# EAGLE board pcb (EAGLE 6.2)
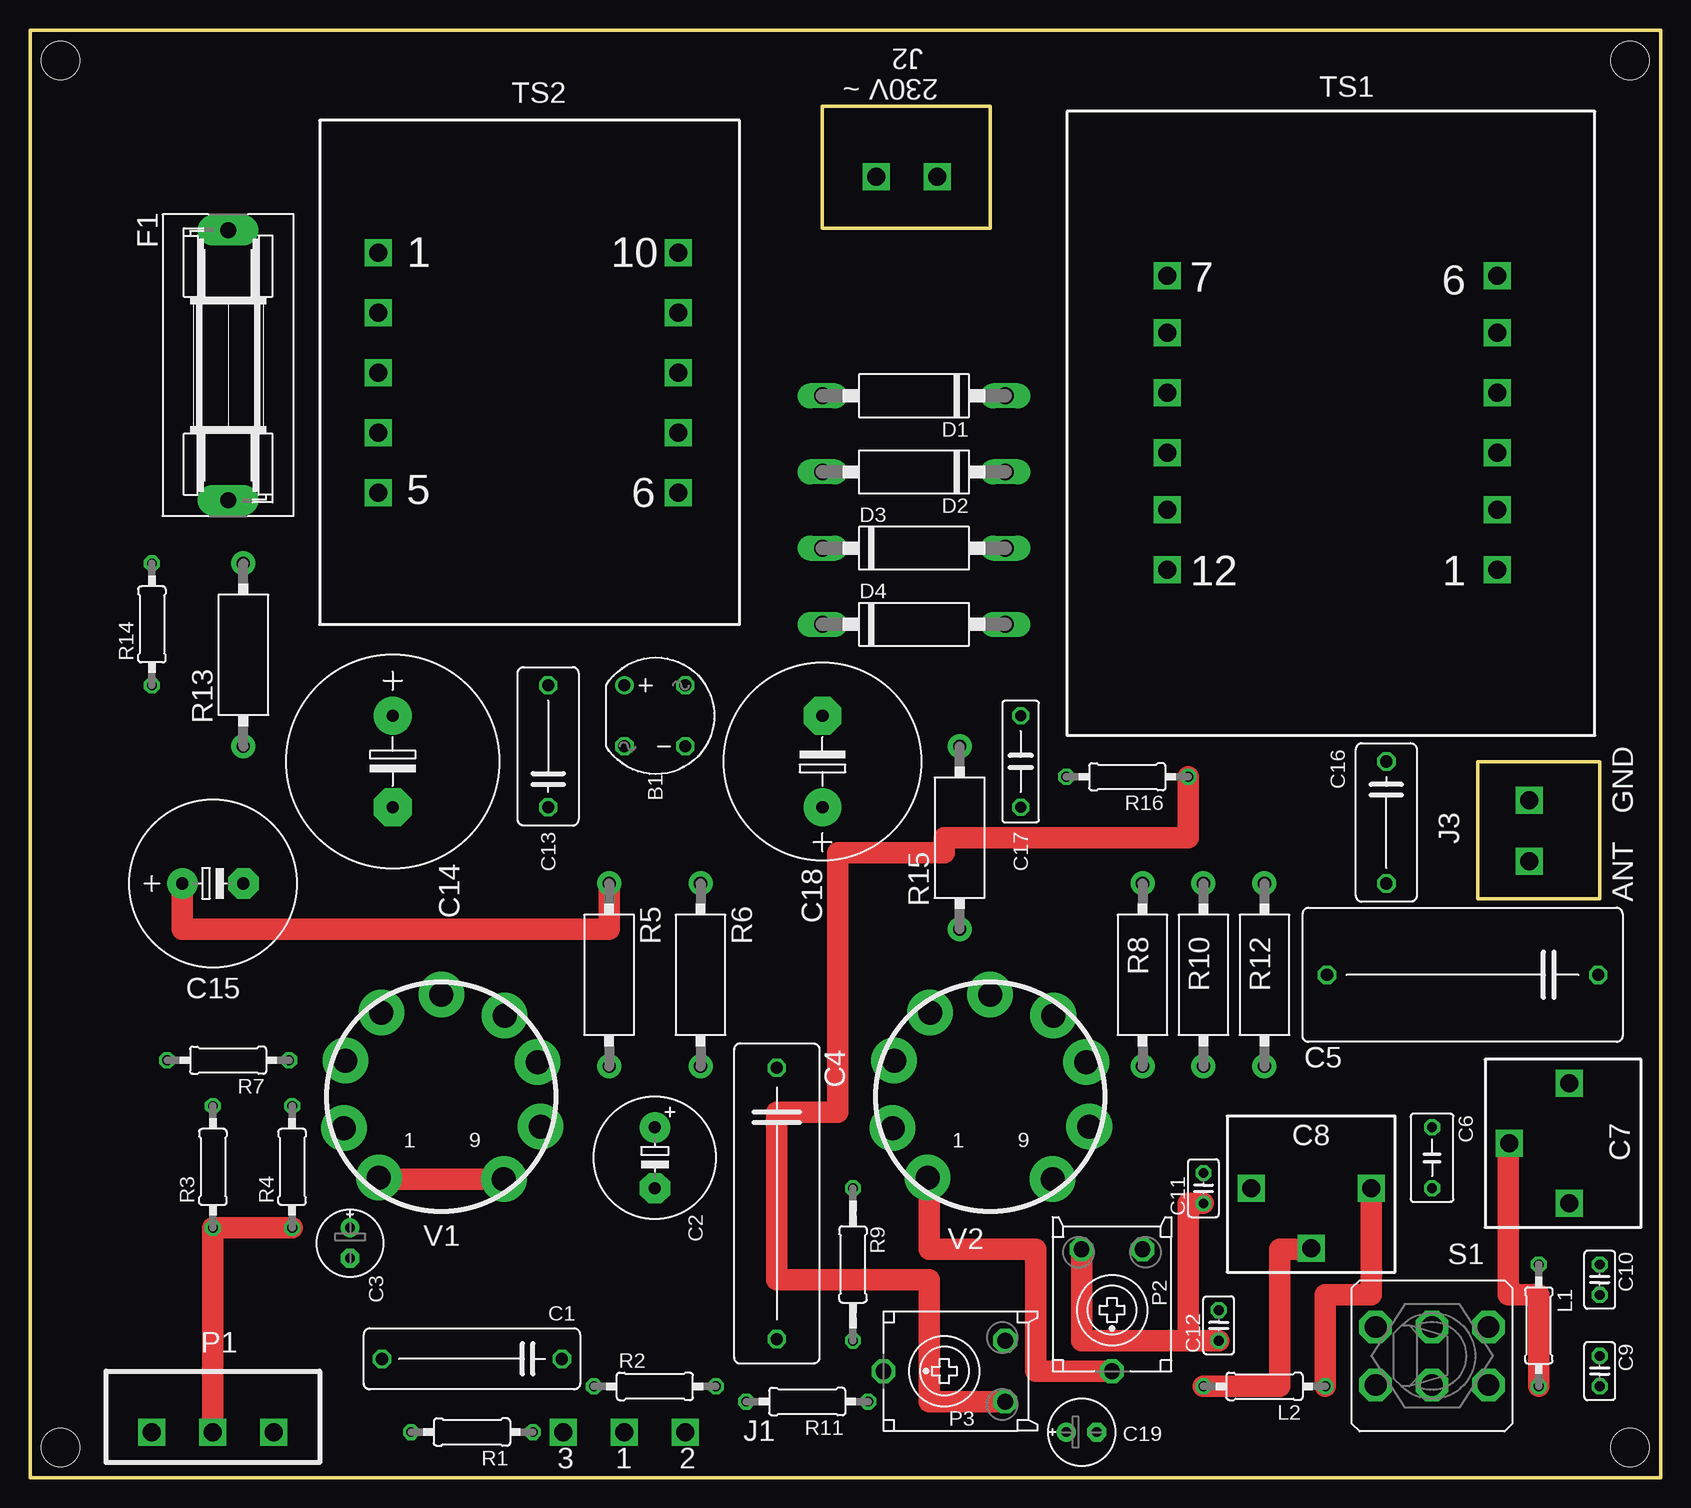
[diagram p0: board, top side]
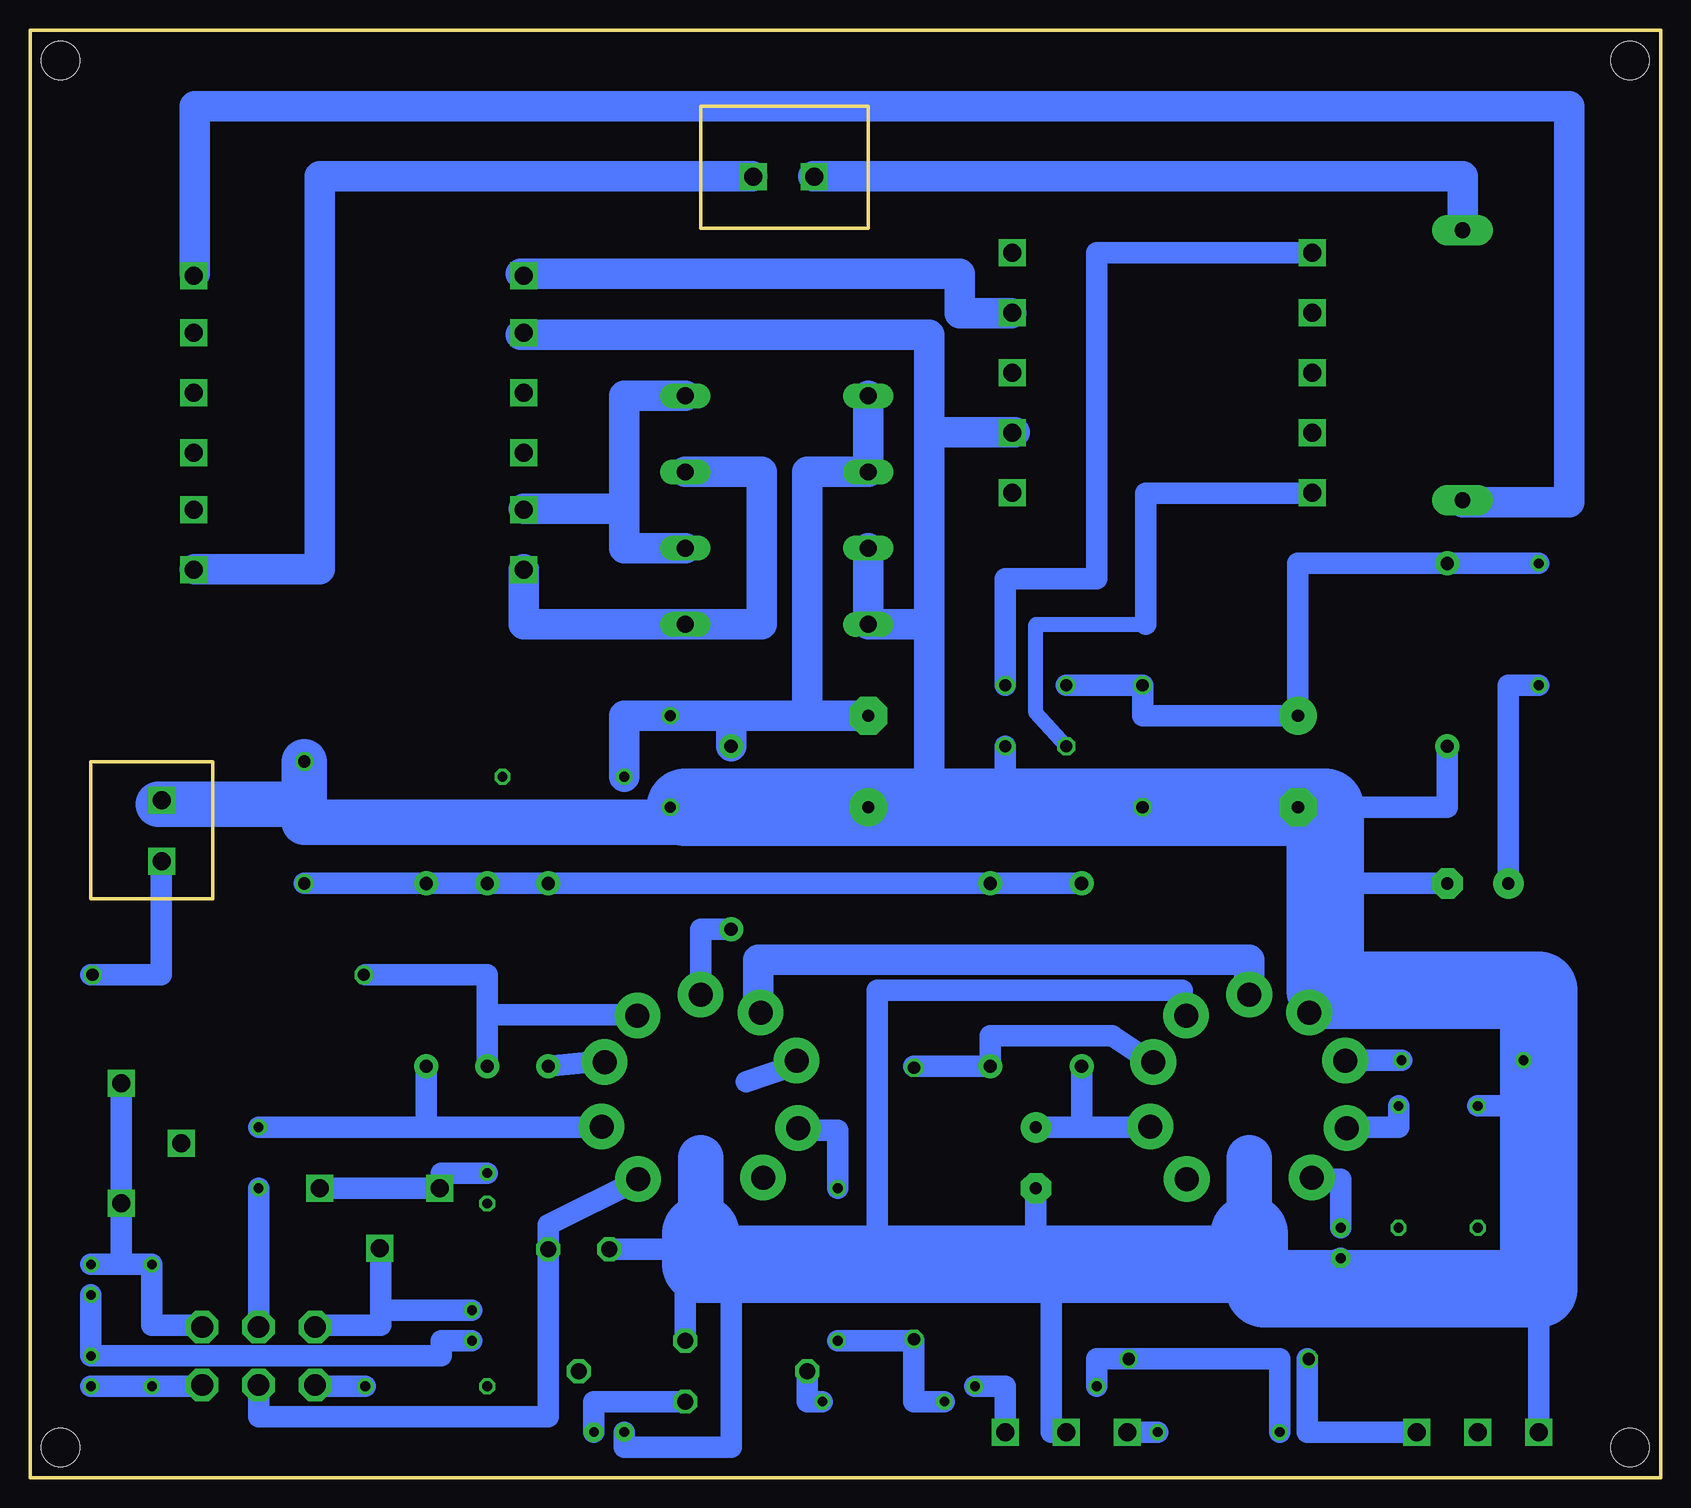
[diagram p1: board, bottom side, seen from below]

Size 135.89 x 120.65 mm. Coordinates in mm from the lower left corner, seen from the top.
Outline: 0,0 135.89,0 135.89,120.65 0,120.65 0,0
Outline: 66.04,104.14 80.01,104.14 80.01,114.3 66.04,114.3 66.04,104.14
Outline: 120.65,59.69 120.65,48.26 130.81,48.26 130.81,59.69 120.65,59.69
Copper layers (1*16): Top 0.035mm / dielectric 1.5mm / Bottom 0.035mm
Design rules: minimum track width 10mil, minimum drill 24mil, track to track 8mil, track to pad 8mil, pad to pad 8mil, via to via 8mil, smd to smd 8mil, copper to edge 40mil, drill to drill 8mil, minimum pad ring 10mil, minimum via ring 8mil, stop-mask expansion 4mil, vias tented up to drill 0mil, thermal gap 10mil
Holes 3.2 mm at 2.54,2.54 133.35,118.11 2.54,118.11 133.35,2.54

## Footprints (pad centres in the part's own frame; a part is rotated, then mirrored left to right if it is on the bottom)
RB1A = drill 1.016: + -2.54,2.54 | drill 1.016 octagon: - 2.54,-2.54; AC1 2.54,2.54; AC2 -2.54,-2.54
C150-054X183 = drill 1.016 octagon: 1 -7.493,0; 2 7.493,0
E5-10,5 = drill 1.016 pad 2.54: + -2.54,0 | drill 1.016 pad 2.54 octagon: - 2.54,0
E2,5-6E = drill 0.813 pad 1.575: + -1.27,0 | drill 0.813 pad 1.575 octagon: - 1.27,0
C225-074X268 = drill 1.016 octagon: 1 -11.303,0; 2 11.303,0
C225-113X268 = drill 1.016 octagon: 1 -11.303,0; 2 11.303,0
C050-035X075 = drill 0.813 octagon: 1 -2.54,0; 2 2.54,0
C025-025X050 = drill 0.813 octagon: 1 -1.27,0; 2 1.27,0
C102-054X133 = drill 1.016 octagon: 1 -5.08,0; 2 5.08,0
E7,5-18 = drill 1.016 pad 3.15: + -3.81,0 | drill 1.016 pad 3.15 octagon: - 3.81,0
E5-13 = drill 1.016 pad 2.54: + -2.54,0 | drill 1.016 pad 2.54 octagon: - 2.54,0
C075-032X103 = drill 0.914 octagon: 1 -3.81,0; 2 3.81,0
E7,5-16 = drill 1.016 pad 3.15: + -3.81,0 | drill 1.016 pad 3.15 octagon: - 3.81,0
C1702E15 = drill 1.397 long: A 7.62,0; C -7.62,0
SH22,5A = drill 1.321 pad 2.54 long: 1 -11.252,0; 2 11.252,0
0207/10 = drill 0.813 octagon: 1 -5.08,0; 2 5.08,0
ECP10S = drill 1.321 octagon: A -2.54,-5.08; E 2.54,-5.08; S 0,5.08
CA0001 = drill 1.1 pad 2: 1 -7.62,0; 2 7.62,0
0207/12 = drill 0.813 octagon: 1 -6.35,0; 2 6.35,0
M9040P2 = drill 1.803 octagon: 1 -2.413,4.699; 2 -2.413,0; 3 -2.413,-4.699; 4 2.413,4.699; 5 2.413,0; 6 2.413,-4.699
NOVAL_OD_STR_DRUKU = drill 2 pad 3.81: 1 5.207,-6.858; 2 8.254,-2.484; 3 8.004,2.893; 4 5.258,6.77; 5 0,8.524; 6 -5.004,7.024; 7 -8.004,3.02; 8 -8.127,-2.611; 9 -5.207,-6.731

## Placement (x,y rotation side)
B1  [RB1A]  52.07,63.5 0 top
C1  [C150-054X183]  36.83,9.91 180 top
C2  [E5-10,5]  52.07,26.67 270 top
C3  [E2,5-6E]  26.67,19.56 270 top
C4  [C225-074X268]  62.23,22.86 270 top
C5  [C225-113X268]  119.38,41.91 180 top
C6  [C050-035X075]  116.84,26.67 270 top
C9  [C025-025X050]  130.81,8.89 270 top
C10  [C025-025X050]  130.81,16.51 270 top
C11  [C025-025X050]  97.79,24.13 90 top
C12  [C025-025X050]  99.06,12.7 90 top
C13  [C102-054X133]  43.18,60.96 90 top
C14  [E7,5-18]  30.23,59.69 270 top
C15  [E5-13]  15.24,49.53 0 top
C16  [C102-054X133]  113.03,54.61 270 top
C17  [C075-032X103]  82.55,59.69 270 top
C18  [E7,5-16]  66.04,59.69 90 top
C19  [E2,5-6E]  87.63,3.81 0 top
D1  [C1702E15]  73.66,90.17 180 top
D2  [C1702E15]  73.66,83.82 180 top
D3  [C1702E15]  73.66,77.47 0 top
D4  [C1702E15]  73.66,71.12 0 top
F1  [SH22,5A]  16.51,92.71 270 top
L1  [0207/10]  125.73,12.7 270 top
L2  [0207/10]  102.87,7.62 180 top
P2  [ECP10S]  90.17,13.97 180 top
P3  [ECP10S]  76.2,8.89 90 top
R1  [0207/10]  36.83,3.81 180 top
R2  [0207/10]  52.07,7.62 0 top
R3  [0207/10]  15.24,25.91 90 top
R4  [0207/10]  21.84,25.91 90 top
R5  [CA0001]  48.26,41.91 270 top
R6  [CA0001]  55.88,41.91 270 top
R7  [0207/10]  16.51,34.8 180 top
R8  [CA0001]  92.71,41.91 270 top
R9  [0207/12]  68.58,17.78 270 top
R10  [CA0001]  97.79,41.91 270 top
R11  [0207/10]  64.77,6.35 180 top
R12  [CA0001]  102.87,41.91 270 top
R13  [CA0001]  17.78,68.58 90 top
R14  [0207/10]  10.16,71.12 90 top
R15  [CA0001]  77.47,53.34 90 top
R16  [0207/10]  91.44,58.42 180 top
S1  [M9040P2]  116.84,10.16 270 top
V1  EF80  [NOVAL_OD_STR_DRUKU]  34.29,31.75 0 top
V2  ECH84  [NOVAL_OD_STR_DRUKU]  80.01,31.75 0 top

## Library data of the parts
B1 = rectifier
C1-C6 C9-C19 L1 L2 R1-R4 R7 R9 R11 R14 R16 = rcl
D1-D4 = diode
F1 = fuse
P2 P3 = pot
R5 R6 R8 R10 R12 R13 R15 = resistor-power
S1 = switch
V1 V2 = tubes

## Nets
S$2: R7.1
S$3: C3.+
S$4: C3.-
S$5: C2.-
S$8: C2.+ R5.2
S$9: R6.2
S$13: B1.- C15.- C17.2 C18.+ D3.C D4.C R13.1
S$15: R1.2 R2.1
S$16: R1.1
S$17: R2.2
S$20: R9.1
S$21: R9.2 R11.2
S$23: R8.2
S$24: R10.2
S$25: C16.1
S$26: P2.A
S$27: P2.S
S$28: L2.2
S$29: P3.S R11.1
S$30: C6.1 R12.2
S$32: C9.1 C10.2 C11.1 C12.1 P2.E P3.E
S$33: C12.2
S$35: C10.1 L1.1
S$36: C11.2 L2.1
S$46: C9.2 L1.2
S$53: R4.2
S$55: R3.2
S$56: R3.1 R4.1
S$84: C17.1 C18.- D1.A D2.A R15.2 R16.2
S$85: D2.C D4.A
S$86: D1.C D3.A
S$87: R15.1
S$89: C19.- P3.A R16.1
S$90: C19.+
S$92: B1.AC1
S$93: B1.AC2
S$95: B1.+ C13.2 C14.+ R13.2 R14.2
S$96: C15.+ C16.2 R5.1 R10.1 R12.1 R14.1

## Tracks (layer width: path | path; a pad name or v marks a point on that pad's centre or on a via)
S$1
  Bottom 3.81: 34.29,20.32 34.29,26.67
  Bottom 6.452: 34.29,20.32 34.29,17.78 80.01,17.78 80.01,20.32
S$2
  Bottom 1.778: R7.1 26.67,34.8
S$3
  Bottom 1.778: C3.+ 26.67,24.89 29.21,24.89
S$4
  Bottom 1.778: C3.- 31.75,16.51
S$5
  Bottom 1.778: 52.07,20.32 C2.-
S$6
  Bottom 1.778: 39.88,38.86 39.88,40.64 65.28,40.64 65.28,17.53
S$7
  Top 1.778: 28.7,24.89 40.13,24.89
S$8
  Bottom 1.778: 48.26,29.21 C2.+ | 41.91,29.21 48.26,29.21 | 48.26,29.21 R5.2
S$9
  Bottom 1.778: 41.91,34.29 45.72,36.83 55.88,36.83 R6.2 62.23,34.29
S$10  (via drill 1.5)
  Bottom 1.778: 50.8,15.24 50.8,3.81 v49.53,3.81
S$11
  Bottom 1.778: 21.84,29.21 26.16,29.21
S$12  (via drill 1.5)
  Bottom 1.778: v20.32,3.81 29.46,3.81 29.46,9.91
S$13  (via drill 1.5)
  Bottom 1.778: 54.61,55.88 B1.- | 29.21,49.53 29.21,39.37 | 29.21,49.53 C15.- | C18.+ 60.96,55.88 | C18.+ 54.61,55.88 | C17.2 81.28,55.88 C18.+ | 29.21,55.88 29.21,49.53 | 29.21,55.88 54.61,55.88 | R13.1 17.78,55.88 27.94,55.88 29.21,55.88 | v10.16,3.81 10.16,14.22 33.02,14.22 33.02,15.75 33.02,16.51
  Bottom 2.54: D3.C D4.C 60.96,71.12 | 60.96,55.88 60.96,71.12 | 60.96,87.12 53.85,87.12 | 95,95.25 60.96,95.25 60.96,71.12
  Bottom 6.452: 81.28,55.88 27.94,55.88 27.94,40.64 10.16,40.64 10.16,15.75 33.02,15.75
S$15
  Bottom 1.778: R2.1 46.99,9.91 31.75,9.91 R1.2
S$16  (via drill 1.5)
  Bottom 1.778: R1.1 v44.45,3.81
S$17  (via drill 1.5)
  Bottom 1.778: R2.2 54.61,7.62 v54.61,3.81
S$18
  Bottom 3.81: 80.01,22.86 80.01,26.67
S$19
  Bottom 1.778: 72.39,34.29 76.2,33.02
S$20
  Bottom 1.778: 71.63,28.96 68.58,28.96 R9.1
S$21
  Bottom 1.778: R9.2 62.23,11.43 62.23,6.35 R11.2
S$22
  Bottom 1.778: 34.29,40.64 34.29,43.18 74.93,43.18 74.93,38.86
S$23
  Bottom 1.778: 87.63,34.8 R8.2
S$24
  Bottom 1.778: 85.09,38.61 97.79,38.61 | 97.79,38.61 R10.2 | 107.95,41.91 97.79,41.91 97.79,38.61
S$25
  Bottom 3.81: 78.74,54.61 113.03,54.61 113.03,56.13 | 113.03,56.13 C16.1 | 113.03,56.13 125.22,56.13
S$26
  Bottom 1.778: 85.09,24.89 92.71,21.08 P2.A 92.71,5.08 116.84,5.08 116.84,7.62
S$27
  Top 1.778: P2.S 83.82,8.89 83.82,19.05 74.93,19.05 74.93,25.15
S$28
  Top 1.778: L2.2 104.14,7.62 104.14,19.05 106.68,19.05
S$29
  Bottom 1.778: R11.1 71.12,6.35 P3.S
S$30
  Bottom 1.778: 102.87,29.21 R12.2 | 88.39,29.21 102.87,29.21 | 102.87,29.21 C6.1
S$31
  Bottom 1.778: 116.84,12.7 116.84,24.13
S$32
  Top 1.778: C11.1 96.52,22.86 96.52,11.43 | 96.52,11.43 C12.1 | 96.52,11.43 87.63,11.43 P2.E
  Bottom 1.778: P2.E 81.28,19.05 P3.E | C12.1 101.6,11.43 101.6,10.16 C9.1 C10.2
S$33
  Bottom 1.778: 106.68,13.97 106.68,19.05 | C12.2 106.68,13.97 | 111.76,12.7 106.68,12.7 106.68,13.97
S$34  (via drill 1.5)
  other vias: 54.03,102.07
S$35
  Bottom 1.778: 121.92,12.7 125.73,12.7 L1.1 128.27,17.78 | 128.27,17.78 C10.1 | 128.27,33.02 128.27,17.78
S$36  (via drill 1.5)
  Top 1.778: v111.76,24.13 111.76,15.24 107.95,15.24 L2.1
  Bottom 1.778: v111.76,24.13 101.6,24.13 101.6,25.4 C11.2 | L2.1 111.76,7.62
S$37  (via drill 1.5)
  other vias: 101.76,24.13
S$38  (via drill 1.5)
  other vias: 106.76,19.13
S$39  (via drill 1.5)
  other vias: 75.62,108.42
S$40  (via drill 1.5)
  other vias: 70.54,108.42
S$41  (via drill 1.5)
  other vias: 124.93,56.46
S$42
  Bottom 1.778: 130.81,41.91 124.97,41.91 124.97,51.31
S$43  (via drill 1.5)
  other vias: 128.27,22.86
S$44  (via drill 1.5)
  other vias: 128.27,32.86
S$45  (via drill 1.5)
  other vias: 123.27,27.86
S$46
  Top 1.778: 123.19,27.94 123.19,15.24 125.73,15.24 L1.2
  Bottom 1.778: 121.92,7.62 L1.2 C9.2
S$47  (via drill 1.5)
  other vias: 124.93,51.38
S$48
  Bottom 2.54: 75.69,108.46 111.76,108.46 111.76,75.69 122.17,75.69
S$49
  Bottom 2.54: 122.17,100.33 122.17,114.3 7.62,114.3 7.62,81.28 16.51,81.28
S$50
  Bottom 2.54: 16.51,104.14 16.51,108.46 70.61,108.46
S$51
  Bottom 2.54: 75.18,38.61 75.18,43.18 34.29,43.18 34.29,40.39
S$52  (via drill 1.5)
  other vias: 29.03,87.07
S$53
  Bottom 1.778: R4.2 21.84,29.46 21.84,29.21
S$55
  Bottom 1.778: R3.2 12.19,30.99
S$56  (via drill 1.5)
  Top 1.778: R4.1 21.59,20.83 R3.1 v15.24,3.81
S$61  (via drill 1.5)
  other vias: 29.03,102.07
S$62  (via drill 1.5)
  other vias: 29.03,97.07
S$63  (via drill 1.5)
  other vias: 29.03,92.07
S$64  (via drill 1.5)
  other vias: 29.03,82.07
S$65  (via drill 1.5)
  other vias: 54.03,82.07
S$66  (via drill 1.5)
  other vias: 54.03,87.07
S$67  (via drill 1.5)
  other vias: 54.03,92.07
S$68  (via drill 1.5)
  other vias: 54.03,97.07
S$69  (via drill 1.5)
  other vias: 122.26,85.42
S$70  (via drill 1.5)
  other vias: 94.76,85.42
S$71  (via drill 1.5)
  other vias: 122.26,75.67
S$72  (via drill 1.5)
  other vias: 122.26,80.67
S$73  (via drill 1.5)
  other vias: 122.26,85.42
S$74  (via drill 1.5)
  other vias: 122.26,90.42
S$75  (via drill 1.5)
  other vias: 122.26,95.42
S$76  (via drill 1.5)
  other vias: 122.26,100.17
S$77  (via drill 1.5)
  other vias: 94.76,100.17
S$78  (via drill 1.5)
  other vias: 94.76,90.42
S$79  (via drill 1.5)
  other vias: 94.76,95.42
S$80  (via drill 1.5)
  other vias: 94.76,85.42
S$81  (via drill 1.5)
  other vias: 94.76,75.67
S$82  (via drill 1.5)
  other vias: 94.76,80.67
S$84
  Bottom 1.778: C18.- 71.12,63.5
  Bottom 2.54: D1.A D2.A 71.12,83.82 71.12,63.5 | 77.47,63.5 C17.1 86.36,63.5 R16.2 | 77.47,63.5 R15.2 | C18.- 77.47,63.5
S$85
  Bottom 2.54: D2.C 74.93,83.82 74.93,71.12 D4.A 94.74,71.12 94.74,75.69
S$86
  Bottom 2.54: D1.C 86.36,90.17 86.36,80.77 | 86.36,80.77 86.36,77.47 D3.A | 86.36,80.77 94.74,80.77
S$87
  Bottom 1.778: R15.1 80.01,45.72 80.01,40.39
S$89
  Top 1.778: P3.A 74.93,6.35 74.93,16.51 62.23,16.51 62.23,30.48 67.31,30.48 67.31,52.07 76.2,52.07 76.2,53.34 96.52,53.34 R16.1
  Bottom 1.778: P3.A 88.9,6.35 C19.-
S$90
  Bottom 1.778: C19.+ 86.36,2.54 77.47,2.54 77.47,15.24
S$91
  Bottom 2.54: 54.1,97.03 58.42,97.03 58.42,100.33 95,100.33
S$92
  Bottom 1.778: 29.21,102.11 46.99,102.11 46.99,74.93 54.61,74.93 B1.AC1
S$93
  Bottom 1.27: 42.93,71.12 52.07,71.12 52.07,63.75 B1.AC2
  Bottom 1.778: 42.93,71.12 42.93,82.04 29.21,82.04
S$95
  Bottom 1.778: B1.+ C13.2 43.18,63.5 C14.+ 30.23,76.2 R13.2 R14.2
S$96
  Top 1.778: R5.1 48.26,45.72 12.7,45.72 C15.+
  Bottom 1.778: C16.2 R12.1 R10.1 R5.1 | R14.1 12.7,66.04 C15.+

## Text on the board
tNames: J2 | 230V ~ | TS2 | TS1 | 1 | 10 | 7 | 6 | 5 | 6 | 12 | 1 | GND | J3 | ANT | C8 | C7 | P1 | J1 | 3 | 1 | 2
